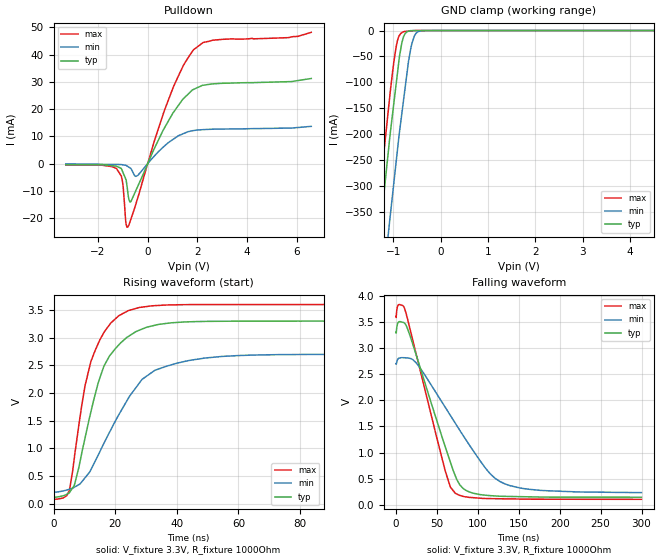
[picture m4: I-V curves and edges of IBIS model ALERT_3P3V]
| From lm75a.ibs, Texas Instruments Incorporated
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|   Model ALERT_3P3V
[Model]   ALERT_3P3V
Model_type   Open_drain
Polarity   Non-Inverting
Vmeas = 1.65
Vref = 3.3
Cref = 15pF
Rref = 1000
|   typ   min   max
|   (nom PVT)   (fast PVT)   (slow PVT)
C_comp   0.576p   0.523p   0.654p
|C_comp (ON state)   0.576p   0.523p   0.654p
|C_comp (OFF state)   0.679p   0.676p   0.701p
| Where   nom PVT is  Nominal Process, 3.3V, 27C
|   Fast PVT is Strong Process, 3.6V, -40C
|   Slow PVT is Weak Process, 2.7V, 150C
[Voltage Range]   3.3   2.7   3.6
[Temperature Range]   27   150   -40
[Pullup Reference]   3.3   2.7   3.6
[Pulldown Reference]   0   0   0
[Power Clamp Reference]   3.3   2.7   3.6
[GND Clamp Reference]   0   0   0
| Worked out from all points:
|   slope of the pulldown table from 0 to 0.495 V, typ, clamps not added: 50.2 ohm
|   GND clamp passes 1 mA (typ) near -0.66 V on its own axis
|   falling waveform, V_fixture 3.3V, R_fixture 1000Ohm: 20-80 % time 38.7ns typ, 61.7ns min, 33.3ns max; typ from 3.3 V to 0.148 V
|   rising waveform, V_fixture 3.3V, R_fixture 1000Ohm: 20-80 % time 9.49ns typ, 15.1ns min, 7.87ns max; typ from 0.145 V to 3.3 V
[Pulldown]
|   Voltage   I(typ)   I(min)   I(max)
-3.3V     -367.1uA   -119uA     -531.5uA
-1.259V   -961.9uA   -335.5uA   -1.787mA
-1.012V   -2.935mA   -446.1uA   -6.844mA
-875.5mV  -5.899mA   -646.1uA   -22.03mA
-804.2mV  -10.37mA   -1.064mA   -23.37mA
-681.5mV  -14.06mA   -1.782mA   -20.53mA
-405.2mV  -8.451mA   -4.399mA   -12.72mA
648.6mV   12.67mA    6.246mA    18.91mA
1.441V    23.85mA    11.01mA    36.13mA
1.837V    27.21mA    12.12mA    41.74mA
2.629V    29.29mA    12.62mA    45.33mA
6.59V     31.27mA    13.68mA    48.23mA
[GND Clamp]
|   Voltage   I(typ)   I(min)   I(max)
-3.3V     -2.268A    -2.367A    -2.221A
-1.457V   -550.3mA   -703.8mA   -472.1mA
-1.271V   -381.5mA   -538.6mA   -301.2mA
-1.073V   -207.5mA   -366.2mA   -128mA
-937.3mV  -102.9mA   -252.9mA   -31.31mA
-867.1mV  -49.43mA   -195.5mA   -9.213mA
-804.2mV  -19.24mA   -150.5mA   -3.065mA
-677.4mV  -1.428mA   -59.86mA   -1.122mA
-603.2mV  -156.9uA   -24.4mA    -518.5uA
-516.6mV  -125uA     -5.11mA    0A
-405.2mV  -83.89uA   -390.3uA   0A
6.59V     0A         0A         0A
[Ramp]
R_load = 1000
|   typ   min   max
dV/dt_r   1.89273/9.49147e-09   1.48063/1.50704e-08   2.09536/7.86528e-09
dV/dt_f   1.89094/3.86447e-08   1.47856/6.16815e-08   2.09527/3.31397e-08
[Falling Waveform]
V_fixture = 3.3V
V_fixture_min = 2.7V
V_fixture_max = 3.6V
R_fixture = 1000Ohm
C_fixture = 0F
|   Time   V(typ)   V(min)   V(max)
0s        3.3V       2.7V       3.6V
3.2ns     3.496V     2.802V     3.828V
10.23ns   3.477V     2.813V     3.765V
24.66ns   2.868V     2.716V     2.884V
60.45ns   1.098V     1.86V      635.4mV
72.45ns   556.9mV    1.562V     224.1mV
90.16ns   245mV      1.133V     144.8mV
114.8ns   178.8mV    600.9mV    121.6mV
132.8ns   164.5mV    404.7mV    117.7mV
299.9ns   148.4mV    235.7mV    107.9mV
[Rising Waveform]
V_fixture = 3.3V
V_fixture_min = 2.7V
V_fixture_max = 3.6V
R_fixture = 1000Ohm
C_fixture = 0F
|   Time   V(typ)   V(min)   V(max)
0s        145.5mV    232.3mV    107.7mV
5.186ns   204.7mV    265.6mV    247.4mV
6.732ns   331.4mV    300.2mV    823.9mV
10.23ns   1.19V      471.1mV    2.136V
15.07ns   2.279V     946.7mV    2.965V
19.93ns   2.794V     1.481V     3.334V
27.83ns   3.135V     2.181V     3.546V
40.34ns   3.277V     2.545V     3.595V
60.79ns   3.299V     2.68V      3.599V
299.9ns   3.3V       2.7V       3.6V
